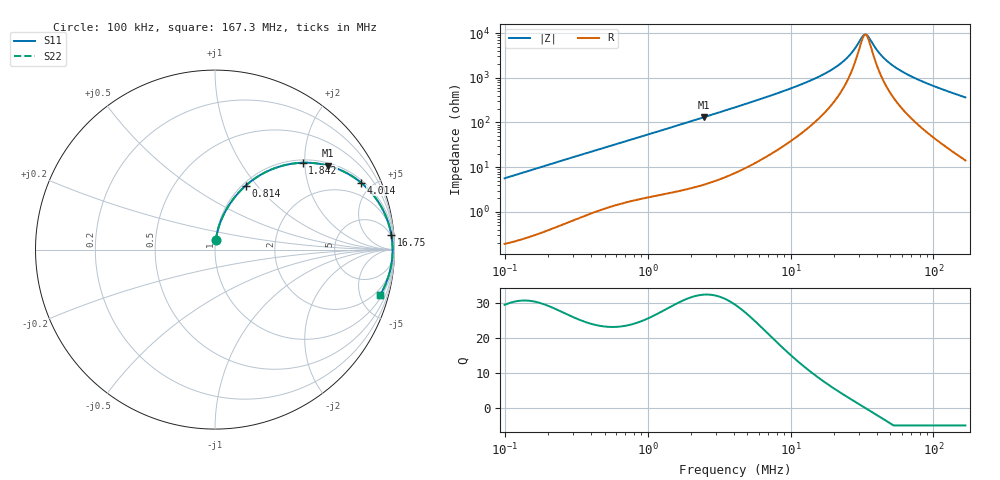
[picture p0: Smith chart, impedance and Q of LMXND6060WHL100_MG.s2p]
! LMXND6060WHL100_MG  S-PARAMETER MODEL  ( General Type )
! Model Generated by TAIYO YUDEN Corporation (http://www.ty-top.com)
! Version 1.0
! TAIYO YUDEN Control No. 191025NI43SB-FBB
! Copyright(c) 2019 TAIYO YUDEN CO.,LTD. All Rights Reserved.
! Product Description (link to TY-COMPAS)
! https://ds.yuden.co.jp/TYCOMPAS/or/detail?pn=LMXND6060WHL100MMG&u=M
! Products Name : Inductors
! Characteristics :
!  Inductance : 10 uH , SRF(min) : 20 MHz , DC Resistance(max) : 0.0845 Ohm
!  Rated Current : Saturation :1900 mA , Temp Rise : 1900 mA
!  Case Size : 6.0 x 6.0 / 0.236 x 0.236 [mm/inch] , Thickness : 2.8 / 0.11 [mm/inch]
!  (Conditions: Temperature = 25 degC , DC Bias Current/Voltage = 0A / 0V)
! External Node Assignments :
!  1  o---GGG---o  2
! GND o---------o GND
! Frequency Range : 0.1MHz  -  167.251077MHz  [ 402 STEP ]
# MHz S RI R 50
! Freq[MHz].  S11 Real  S11 Imag  S21 Real  S21 Imag  S12 Real  S12 Imag  S22 Real  S22 Imag
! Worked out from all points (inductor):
!   401 points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, 100 kHz to 167.3 MHz, reference 50 ohm
!   read as one part in series: L = 8.95 uH near 103.8 kHz
!   highest Q = 32.3 at 2.478 MHz (marker M1), where L = 8.42 uH
!   self-resonance near 33.29 MHz
!   S11 on the Smith chart (normalised r, x): 100 kHz: 1.00, +0.11; 814 kHz: 1.04, +0.87; 1.842 MHz: 1.06, +1.95; 4.014 MHz: 1.14, +4.28; 16.75 MHz: 4, +23; 167.3 MHz: 1.28, -7.28
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0.1  0.00506 0.0559  0.9949 -0.0559  0.9949 -0.0559  0.00506 0.0559
0.346668  0.0423 0.1822  0.9577 -0.1822  0.9577 -0.1822  0.0423 0.1822
0.813957  0.1709 0.3562  0.8291 -0.3562  0.8291 -0.3562  0.1709 0.3562
1.20179  0.2973 0.439  0.7027 -0.439  0.7027 -0.439  0.2973 0.439
1.841502  0.4879 0.484  0.5121 -0.484  0.5121 -0.484  0.4879 0.484
2.478033  0.6287 0.4679  0.3713 -0.4679  0.3713 -0.4679  0.6287 0.4679
4.01445  0.8126 0.3737  0.1874 -0.3737  0.1874 -0.3737  0.8126 0.3737
4.166227  0.8234 0.3646  0.1766 -0.3646  0.1766 -0.3646  0.8234 0.3646
7.004525  0.9267 0.238  0.0733 -0.238  0.0733 -0.238  0.9267 0.238
14.17747  0.9775 0.1065  0.0225 -0.1065  0.0225 -0.1065  0.9775 0.1065
16.75423  0.9822 0.0827  0.0178 -0.0827  0.0178 -0.0827  0.9822 0.0827
20.54789  0.9861 0.0562  0.0139 -0.0562  0.0139 -0.0562  0.9861 0.0562
24.28248  0.988 0.0361  0.012 -0.0361  0.012 -0.0361  0.988 0.0361
27.65043  0.9889 0.0212  0.0111 -0.0212  0.0111 -0.0212  0.9889 0.0212
31.48552  0.9893 0.00658  0.0107 -0.00658  0.0107 -0.00658  0.9893 0.00658
33.28788  0.9894 0.000354  0.0106 -0.000354  0.0106 -0.000354  0.9894 0.000354
35.19342  0.9894 -0.00587  0.0106 0.00587  0.0106 0.00587  0.9894 -0.00587
41.58984  0.9888 -0.0247  0.0112 0.0247  0.0112 0.0247  0.9888 -0.0247
49.14881  0.9875 -0.0442  0.0125 0.0442  0.0125 0.0442  0.9875 -0.0442
60.27756  0.9845 -0.0696  0.0155 0.0696  0.0155 0.0696  0.9845 -0.0696
78.15803  0.978 -0.1057  0.022 0.1057  0.022 0.1057  0.978 -0.1057
167.2511  0.9215 -0.2502  0.0785 0.2502  0.0785 0.2502  0.9215 -0.2502
